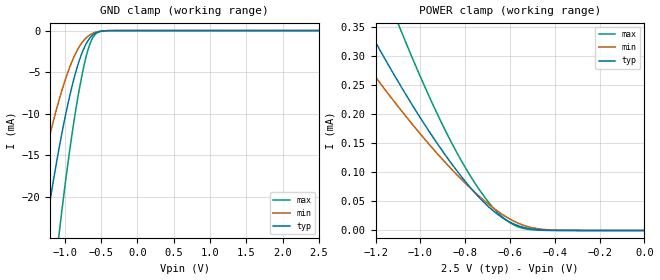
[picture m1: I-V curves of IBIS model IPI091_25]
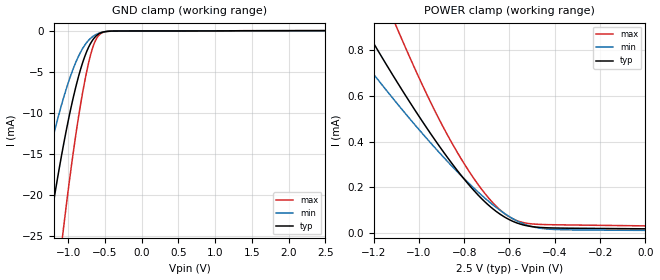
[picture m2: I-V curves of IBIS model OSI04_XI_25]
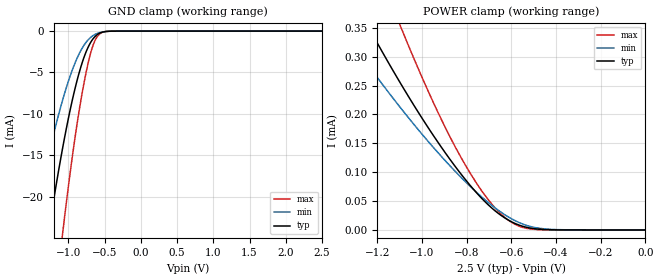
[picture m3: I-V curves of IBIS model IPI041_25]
| TEXAS INSTRUMENTS INCORPORATED
| Connectivity Solutions Group
| IBIS Model of TL16CP754CPM_2.5V
| P754C_PM_2.5V
| This file contains package information for the following:
|  QFP 64-pin (QFP) package as [Component] P754CPM_2.5V
| This device can be powered at the following Vccs:
|  2.5 Volt Vcc
| This file provides unique models under the [Model Selector] for each Vcc.
| For operation at a specific Vcc, select the appropriate model after each
| [Model Selector] keyword.
[IBIS Ver]   3.2
[Comment char]  |_char
[File Name]   P754C_PM_2.5V.ibs
[File Rev]   1 | a
[Date]   December 5, 2007
[Source]   Data created from TI-SPICE simulations at TI-CONN.
[Notes]   The following is an IBIS list for the P754C_PM_2.5V.
   Please contact s-ly@ti.com with questions and
   comments concerning CONN IBIS models.
[Disclaimer] Property of Texas Instruments Incorporated.  Unauthorized
   reproduction and/or distribution is strictly prohibited.
   This product is protected under copyright law.
   Created  2003, (C) Copyright  2003, Texas Instruments
   Incorporated, All Rights Reserved
   UNLESS THERE IS A SIGNED, WRITTEN AGREEMENT TO THE
   CONTRARY, TEXAS INSTRUMENTS (TI) IS PROVIDING THE IBIS
   MODELS  AND WITHOUT ANY WARRANTY, EXPRESSED OR
   IMPLIED.  TI assumes no liability for:
   1) the accuracy of the IBIS models provided to your
   company;
   2) the proper functioning of these IBIS Models in your
   design or for any resulting applications; or
   3) infringement of patents, copyrights or intellectual
   property rights resulting from your use of these IBIS
   models.
   TI provides IBIS Models as a service to our customers.
   You and your company shall not distribute, sell or give
   these models to anyone else without prior written
   permission from TI.
   TI reserves the right to make changes to our products or
   to discontinue any semiconductor product or service
   without notice, and advises our customers to obtain the
   latest version of relevant information to verify, before
   placing orders, that the information being relied on is
   current.
   Please be aware that your receipt and use of the IBIS
   information provided shall serve as acceptance of these
   terms and conditions.  If you do not accept these terms,
   you should return or destroy the IBIS models and any
   other accompanying information immediately.
| Component P754C_2.5V_QFP 64-pin QFP
[Component]   P754C_PM_2.5V
[Manufacturer]   Texas Instruments, Inc.
[Package]
|   typ   min   max
R_pkg   0.03387   0.03002   0.03772
L_pkg   2.23674n   1.83543n   2.63805n
C_pkg   0.53952p   0.46196p   0.61708p
[Pin]   signal_name   model_name   R_pin   L_pin   C_pin
1   DSRA   IPI041   0.03729   2.63770n   0.54873p
2   CTSA   IPI041   0.03373   2.35631n   0.61212p
3   DTRA   OPJ430   0.03280   2.22331n   0.58366p
4   VCC   POWER   0.03224   2.13122n   0.55769p
5   RTSA   OPJ430   0.03153   2.03432n   0.53110p
6   INTA   OPJ430   0.03117   1.96768n   0.51149p
7   CSA   IPI041   0.03104   1.92183n   0.49798p
8   TXA   OPJ430   0.03010   1.83593n   0.46505p
9   IOW   IPI041   0.03007   1.83565n   0.46474p
10   TXB   OPJ430   0.03096   1.92107n   0.49718p
11   CSB   IPI041   0.03110   1.96691n   0.51031p
12   INTB   OPJ430   0.03159   2.04484n   0.53228p
13   RTSB   OPJ430   0.03190   2.11324n   0.55339p
14   GND   GND   0.03265   2.22076n   0.58208p
15   DTRB   OPJ430   0.03352   2.34940n   0.60960p
16   CTSB   IPI041   0.03704   2.62435n   0.54475p
17   DSRB   IPI041   0.03652   2.61027n   0.54700p
18   CDB   IPI041   0.03354   2.34759n   0.61094p
19   RIB   IPI041   0.03281   2.22592n   0.58639p
20   RXB   IPI041   0.03222   2.12197n   0.55702p
21   CLKSEL   IPI041   0.03176   2.03735n   0.53446p
22   A2   IPI041   0.03147   1.97163n   0.51867p
23   A1   IPI041   0.03142   1.92513n   0.50753p
24   A0   IPI041   0.03060   1.83543n   0.47574p
25   XTAL1   OSI04_XI   0.03077   1.83703n   0.47632p
26   XTAL2   OSI04   0.03175   1.92839n   0.50935p
27   RESET   IPI091   0.03188   1.96764n   0.51741p
28   GND   GND   0.03231   2.03651n   0.53599p
29   RXC   IPI041   0.03305   2.13263n   0.56045p
30   RIC   IPI041   0.03384   2.23892n   0.58782p
31   CDC   IPI041   0.03485   2.37358n   0.61708p
32   DSRC   IPI041   0.03772   2.62774n   0.54992p
33   CTSC   IPI041   0.03656   2.61266n   0.54247p
34   DTRC   OPJ430   0.03318   2.35035n   0.60872p
35   VCC   POWER   0.03220   2.20948n   0.57926p
36   RTSC   OPJ430   0.03156   2.10738n   0.55066p
37   INTC   OPJ430   0.03109   2.02413n   0.52649p
38   CSC   IPI041   0.03082   1.95908n   0.50691p
39   TXC   OPJ430   0.03074   1.91419n   0.49349p
40   IOR   IPI041   0.03002   1.83657n   0.46196p
41   TXD   OPJ430   0.03011   1.83744n   0.46243p
42   CSD   IPI041   0.03111   1.92648n   0.49841p
43   INTD   OPJ430   0.03138   1.98201n   0.51625p
44   RTSD   OPJ430   0.03165   2.03099n   0.52844p
45   GND   GND   0.03234   2.12591n   0.55667p
46   DTRD   OPJ430   0.03314   2.23103n   0.58547p
47   CTSD   IPI041   0.03404   2.35574n   0.61001p
48   DSRD   IPI041   0.03771   2.63805n   0.54698p
49   CDD   IPI041   0.03740   2.63294n   0.54729p
50   RID   IPI041   0.03400   2.36300n   0.61328p
51   RXD   IPI041   0.03308   2.22978n   0.58494p
52   VCC   POWER   0.03236   2.12568n   0.55651p
53   D0   IPI04_OPJ43   0.03191   2.05000n   0.53623p
54   D1   IPI04_OPJ43   0.03138   1.96454n   0.50911p
55   D2   IPI04_OPJ43   0.03132   1.92758n   0.49950p
56   D3   IPI04_OPJ43   0.03043   1.84011n   0.46416p
57   D4   IPI04_OPJ43   0.03039   1.83956n   0.46402p
58   D5   IPI04_OPJ43   0.03129   1.92740n   0.49881p
59   D6   IPI04_OPJ43   0.03132   1.96376n   0.50826p
60   D7   IPI04_OPJ43   0.03166   2.03022n   0.52764p
61   GND   GND   0.03226   2.12401n   0.55545p
62   RXA   IPI041   0.03290   2.21862n   0.57989p
63   RIA   IPI041   0.03389   2.36071n   0.61163p
64   CDA   IPI041   0.03726   2.62194n   0.54302p
| Model IPI091
[Model Selector]   IPI091
IPI091_25   2.5 volt Vcc
| Model OSI04_XI
[Model Selector]   OSI04_XI
OSI04_XI_25   2.5 volt Vcc
| Model IPI041
[Model Selector]   IPI041
IPI041_25   2.5 volt Vcc
| Model IPI04_OPJ43
[Model Selector]   IPI04_OPJ43
IPI04_OPJ43_25   2.5 volt Vcc
| Model OPJ430
[Model Selector]   OPJ430
OPJ430_25   2.5 volt Vcc
| Model OSI04
[Model Selector]   OSI04
OSI04_25   2.5 volt Vcc
| Models and submodels in the file (6): IPI091_25 (Input), OSI04_XI_25 (Input), IPI041_25 (Input), IPI04_OPJ43_25 (I/O), OPJ430_25 (3-state), OSI04_25 (3-state)
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[Model]   IPI091_25
Model_type  Input
Vinl = 0
Vinh = 2.5
| variable   typ   min   max
C_comp   1.09pF   0.97pF   1.21pF
[Temperature Range]   40   125   -40
| Ambient temperature   25   110   -40
[Voltage range]   2.5   2.3   2.7
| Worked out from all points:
|   GND clamp passes 1 mA (typ) near -0.66 V on its own axis
|   POWER clamp passes 1 mA (typ) near -2.03 V on its own axis
[GND Clamp]
| IPI091_25
|   Voltage   I(typ)   I(min)   I(max)
-2.5V     -115mA     -79.72mA   -164.4mA
-1.485V   -37.43mA   -23.94mA   -59.12mA
-1.265V   -23.92mA   -14.77mA   -39.38mA
-1.08V    -14.2mA    -8.377mA   -24.56mA
-1.065V   -13.5mA    -7.923mA   -23.45mA
-955mV    -8.737mA   -4.937mA   -15.83mA
-830mV    -4.417mA   -2.392mA   -8.532mA
-730mV    -2.005mA   -1.091mA   -3.99mA
-635mV    -690.9uA   -415.3uA   -1.203mA
-560mV    -221.4uA   -161.8uA   -300.1uA
-440mV    -21.14uA   -26.42uA   -19.38uA
2.5V      179.9pA    7.156nA    49.54pA
[POWER Clamp]
| IPI091_25
|   Voltage   I(typ)   I(min)   I(max)
-2.5V     1.454mA    1.097mA    2.083mA
-1.36V    439.4uA    350.2uA    624.8uA
-1.235V   348.4uA    282.4uA    491.3uA
-1.095V   253.5uA    211.2uA    352uA
-1.075V   240.6uA    201.5uA    333.1uA
-945mV    161.4uA    141.3uA    217.5uA
-830mV    99.28uA    93.13uA    129uA
-720mV    49.87uA    53.05uA    61.07uA
-630mV    21.07uA    26.64uA    21.99uA
-550mV    6.466uA    10.43uA    4.583uA
-465mV    1.046uA    2.442uA    370.2nA
-31.11fV  179.9pA    1.684nA    54.24pA
[Model]   OSI04_XI_25
Model_type  Input
Vinl = 0
Vinh = 2.5
| variable   typ   min   max
C_comp   1.81pF   1.12pF   2.40pF
[Temperature Range]   40   125   -40
| Ambient temperature   25   110   -40
[Voltage range]   2.5   2.3   2.7
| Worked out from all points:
|   GND clamp passes 1 mA (typ) near -0.66 V on its own axis
|   POWER clamp passes 1 mA (typ) near -1.30 V on its own axis
[GND Clamp]
| OSI04_XI_25
|   Voltage   I(typ)   I(min)   I(max)
-2.5V     -117.2mA   -81mA      -167.9mA
-1.48V    -38.04mA   -24.27mA   -60.11mA
-1.26V    -24.32mA   -15mA      -40.01mA
-1.075V   -14.44mA   -8.535mA   -24.92mA
-1.06V    -13.72mA   -8.076mA   -23.8mA
-930mV    -8.097mA   -4.582mA   -14.76mA
-815mV    -4.206mA   -2.33mA    -8.111mA
-710mV    -1.776mA   -1.037mA   -3.434mA
-625mV    -669.3uA   -465.2uA   -1.116mA
-545mV    -205.3uA   -194.2uA   -270.4uA
-430mV    -40.49uA   -47uA      -53.13uA
2.5V      19.05uA    13.35uA    29.56uA
[POWER Clamp]
| OSI04_XI_25
|   Voltage   I(typ)   I(min)   I(max)
-2.5V     3.431mA    2.617mA    4.916mA
-1.355V   1.099mA    896.3uA    1.535mA
-1.24V    898.6uA    746.4uA    1.242mA
-1.22V    864.6uA    720.9uA    1.193mA
-1.095V   659.2uA    565.9uA    893.7uA
-935mV    416.4uA    380.2uA    546.2uA
-830mV    273.7uA    268.3uA    352.9uA
-720mV    148uA      163.2uA    188uA
-625mV    72.54uA    88.13uA    88.07uA
-555mV    40.52uA    47.83uA    50.59uA
-465mV    25.13uA    21.75uA    38.3uA
-31.11fV  19.05uA    12.27uA    31.94uA
[Model]   IPI041_25
Model_type  Input
Vinl = 0
Vinh = 2.5
| variable   typ   min   max
C_comp   1.10pF   0.98pF   1.21pF
[Temperature Range]   40   125   -40
| Ambient temperature   25   110   -40
[Voltage range]   2.5   2.3   2.7
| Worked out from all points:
|   GND clamp passes 1 mA (typ) near -0.66 V on its own axis
|   POWER clamp passes 1 mA (typ) near -2.03 V on its own axis
[GND Clamp]
| IPI041_25
|   Voltage   I(typ)   I(min)   I(max)
-2.5V     -115mA     -79.72mA   -164.4mA
-1.485V   -37.43mA   -23.94mA   -59.12mA
-1.265V   -23.92mA   -14.77mA   -39.38mA
-1.08V    -14.2mA    -8.377mA   -24.56mA
-1.065V   -13.5mA    -7.923mA   -23.45mA
-955mV    -8.737mA   -4.937mA   -15.83mA
-830mV    -4.417mA   -2.392mA   -8.532mA
-730mV    -2.005mA   -1.091mA   -3.99mA
-635mV    -690.9uA   -415.3uA   -1.203mA
-560mV    -221.4uA   -161.8uA   -300.1uA
-440mV    -21.14uA   -26.42uA   -19.38uA
2.5V      179.9pA    7.156nA    49.54pA
[POWER Clamp]
| IPI041_25
|   Voltage   I(typ)   I(min)   I(max)
-2.5V     1.454mA    1.097mA    2.083mA
-1.36V    439.4uA    350.2uA    624.8uA
-1.235V   348.4uA    282.4uA    491.3uA
-1.095V   253.5uA    211.2uA    352uA
-1.075V   240.6uA    201.5uA    333.1uA
-945mV    161.4uA    141.3uA    217.5uA
-830mV    99.28uA    93.13uA    129uA
-720mV    49.87uA    53.05uA    61.07uA
-630mV    21.07uA    26.64uA    21.99uA
-550mV    6.466uA    10.43uA    4.583uA
-465mV    1.046uA    2.442uA    370.2nA
-31.11fV  179.9pA    1.684nA    54.24pA
